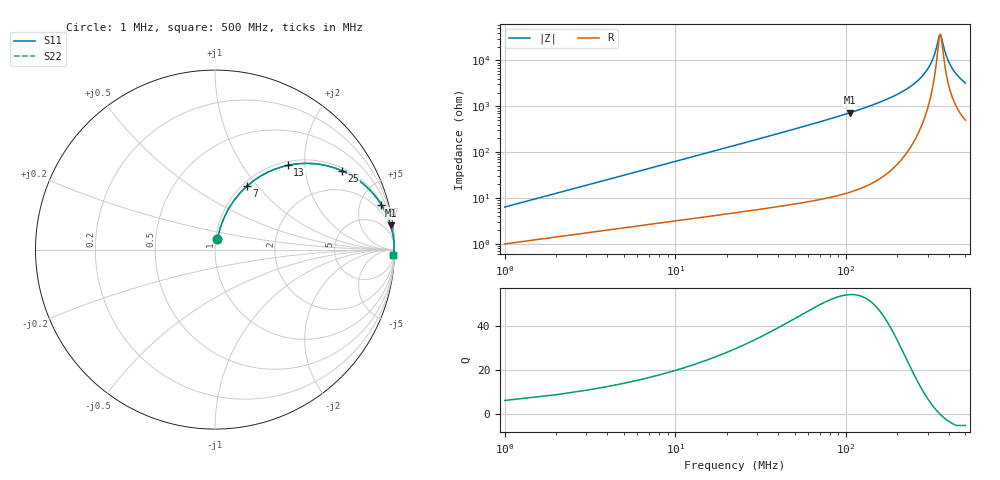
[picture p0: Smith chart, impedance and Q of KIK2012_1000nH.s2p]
!version-2
!date-01.2022
!Series
# MHz S RI R 50
!Freq ReS11 ImS11 ReS21 ImS21 ReS12 ImS12 ReS22 ImS22
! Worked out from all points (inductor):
!   500 points, 1 MHz to 500 MHz, reference 50 ohm
!   read as one part in series: L = 1 uH near 3 MHz
!   highest Q = 54.1 at 105 MHz (marker M1), where L = 1.1 uH
!   self-resonance near 356 MHz
!   S11 on the Smith chart (normalised r, x): 1 MHz: 1.02, +0.13; 7 MHz: 1.05, +0.88; 13 MHz: 1.07, +1.64; 25 MHz: 1.10, +3.16; 57 MHz: 1.16, +7.35; 500 MHz: 11, -64
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1  0.0137 0.0614  0.9863 -0.0614  0.9863 -0.0614  0.0137 0.0614
4  0.0757 0.2278  0.9243 -0.2278  0.9243 -0.2278  0.0757 0.2278
7  0.177 0.3528  0.823 -0.3528  0.823 -0.3528  0.177 0.3528
10  0.2933 0.4308  0.7067 -0.4308  0.7067 -0.4308  0.2933 0.4308
13  0.4054 0.4694  0.5946 -0.4694  0.5946 -0.4694  0.4054 0.4694
19  0.5863 0.4745  0.4137 -0.4745  0.4137 -0.4745  0.5863 0.4745
25  0.7078 0.439  0.2922 -0.439  0.2922 -0.439  0.7078 0.439
38  0.8473 0.3468  0.1527 -0.3468  0.1527 -0.3468  0.8473 0.3468
57  0.9264 0.2504  0.0736 -0.2504  0.0736 -0.2504  0.9264 0.2504
85  0.9667 0.1701  0.0333 -0.1701  0.0333 -0.1701  0.9667 0.1701
105  0.9788 0.1351  0.0212 -0.1351  0.0212 -0.1351  0.9788 0.1351
168  0.993 0.073  0.00704 -0.073  0.00704 -0.073  0.993 0.073
251  0.9972 0.0318  0.00281 -0.0318  0.00281 -0.0318  0.9972 0.0318
302  0.9976 0.0148  0.00238 -0.0148  0.00238 -0.0148  0.9976 0.0148
320  0.9976 0.00956  0.00241 -0.00956  0.00241 -0.00956  0.9976 0.00956
334  0.9975 0.00575  0.0025 -0.00575  0.0025 -0.00575  0.9975 0.00575
351  0.9974 0.00134  0.00265 -0.00134  0.00265 -0.00134  0.9974 0.00134
357  0.9973 -0.00016  0.00271 0.00016  0.00271 0.00016  0.9973 -0.00016
387  0.9969 -0.00731  0.00313 0.00731  0.00313 0.00731  0.9969 -0.00731
417  0.9963 -0.0139  0.00368 0.0139  0.00368 0.0139  0.9963 -0.0139
453  0.9955 -0.0214  0.00448 0.0214  0.00448 0.0214  0.9955 -0.0214
500  0.9943 -0.0303  0.00572 0.0303  0.00572 0.0303  0.9943 -0.0303
